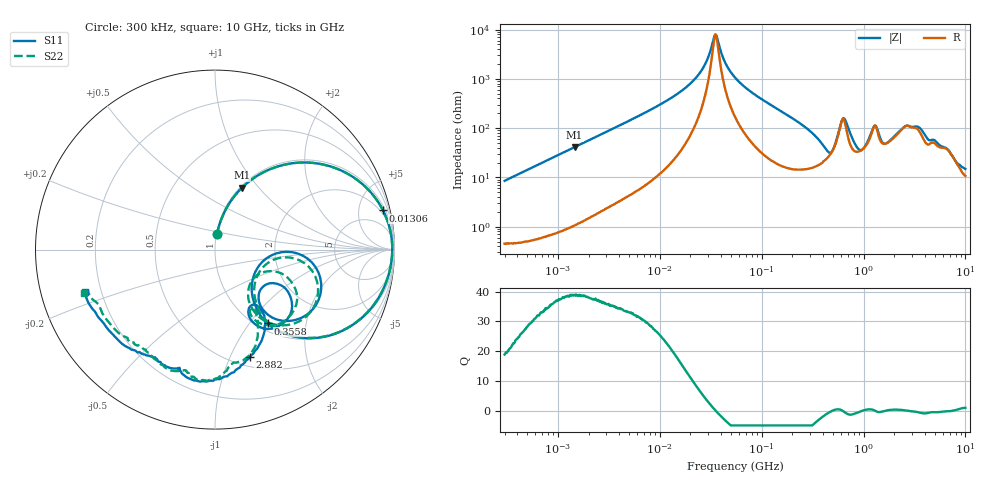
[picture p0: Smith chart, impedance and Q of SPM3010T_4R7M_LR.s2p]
! S-Parameter Data Generated by TDK Corporation
! Copyright(C) 2019 TDK Corporation.
! All Rights Reserved.
! TDK P/N: SPM3010T-4R7M-LR (Inductor)
! Property: L=4.7uH at 100kHz
! Size(LxWxT): 3.2x3x1mm
! Model Type: s2p (Touchstone File Format Version 1.0)
! Frequency: DC=Yes Start=0.3MHz Stop=10000MHz 802points Log-sweep
! Model Generated on Sep. 23, 2019
! Port Assignments:
!  1 ---@@@--- 2
! Applicable Conditions:
!  Temperature = 25 degC
!  DC Bias Current = 0 A
!  Small Signal Operation
! Terms and conditions regarding TDK Simulation Models
! (1)This simulation model is being provided solely for informational purposes. Please refer to the specifications of the products in terms of detailed characteristics of such products.
! (2)In no event shall TDK Corporation of any of its subsidiaries be liable for any loss or damage arising, directly or indirectly,
!  From any information contained in this simulation model, including, but not limited to loss or damages arising from any inaccuracies, omissions or errors in connection with such information.
! (3)Any and all copyrights on this simulation model are owned by TDK Corporation.
!  Duplication or redistribution of this simulation model without prior written permission from TDK Corporation is prohibited.
! (4)This simulation model is subject to any modification or change without any prior notice.
! (5)Neither TDK Corporation nor any of its subsidiaries shall make any warranty, express or implied,
!  Including but not limited to the correctness, implied warranties of merchantability and fitness for a particular purpose with respect to this simulation models.
! (6)The use of this simulation model shall be deemed to have consented to the terms and conditions hereof.
# Hz S MA R 50
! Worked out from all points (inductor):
!   801 points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, 300 kHz to 10 GHz, reference 50 ohm
!   read as one part in series: L = 4.51 uH near 318.3 kHz
!   highest Q = 38.9 at 1.457 MHz (marker M1), where L = 4.49 uH
!   self-resonance near 35.12 MHz
!   S11 on the Smith chart (normalised r, x): 300 kHz: 1.01, +0.17; 13.06 MHz: 1.46, +8.46; 355.8 MHz: 1.12, -1.24; 2.882 GHz: 0.60, -1.19; 10 GHz: 0.14, -0.16
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300000  0.08604 82.3  0.9916 -4.8  0.9914 -4.8  0.08582 82.5
1456635  0.3769 66.4  0.9166 -22.1  0.9166 -22.1  0.3769 66.4
1713600  0.4307 63.0  0.8914 -25.5  0.8913 -25.5  0.4306 63.0
3866967  0.7252 41.8  0.6676 -46.5  0.6678 -46.5  0.7252 41.8
9671944  0.9332 18.8  0.3253 -69.0  0.3255 -69.0  0.933 18.8
1.306337e7  0.9615 13.1  0.2319 -74.1  0.2321 -74.1  0.9613 13.1
2.473055e7  0.986 3.7  0.07467 -77.7  0.07476 -77.7  0.9859 3.7
3.511624e7  0.9875 -0.7  0.01241 -5.9  0.01243 -5.8  0.9874 -0.7
5.477226e7  0.9811 -6.5  0.09202 74.4  0.09207 74.4  0.9809 -6.5
1.405283e8  0.907 -24.2  0.3585 61.5  0.3586 61.5  0.9067 -24.1
3.126428e8  0.6028 -50.6  0.6951 29.2  0.6954 29.1  0.6028 -50.3
3.558009e8  0.5066 -54.4  0.7404 21.1  0.7407 21.1  0.508 -53.7
4.807079e8  0.2591 -32.7  0.7526 -3.5  0.7529 -3.5  0.2775 -32.1
5.497689e8  0.3707 -2.2  0.6204 -17.6  0.6207 -17.7  0.3905 -6.3
6.325141e8  0.6219 -17.9  0.3795 -4.8  0.3796 -4.8  0.6233 -22.9
7.235338e8  0.5855 -42.4  0.559 13.0  0.5593 13.0  0.5671 -48.1
1.001841e9  0.3372 -39.3  0.6999 -16.2  0.7002 -16.3  0.2695 -40.4
1.292013e9  0.5542 -41.0  0.441 -22.8  0.4411 -22.9  0.5348 -31.1
1.767019e9  0.3737 -55.1  0.5985 -31.0  0.5987 -31.0  0.3863 -58.7
2.882439e9  0.6303 -72.2  0.3703 -41.4  0.3704 -41.5  0.6402 -78.8
5.157474e9  0.7051 -112.1  0.3972 -50.2  0.3971 -50.2  0.7169 -109.8
1e10  0.7642 -161.8  0.3219 -95.4  0.3226 -95.6  0.7705 -161.6
